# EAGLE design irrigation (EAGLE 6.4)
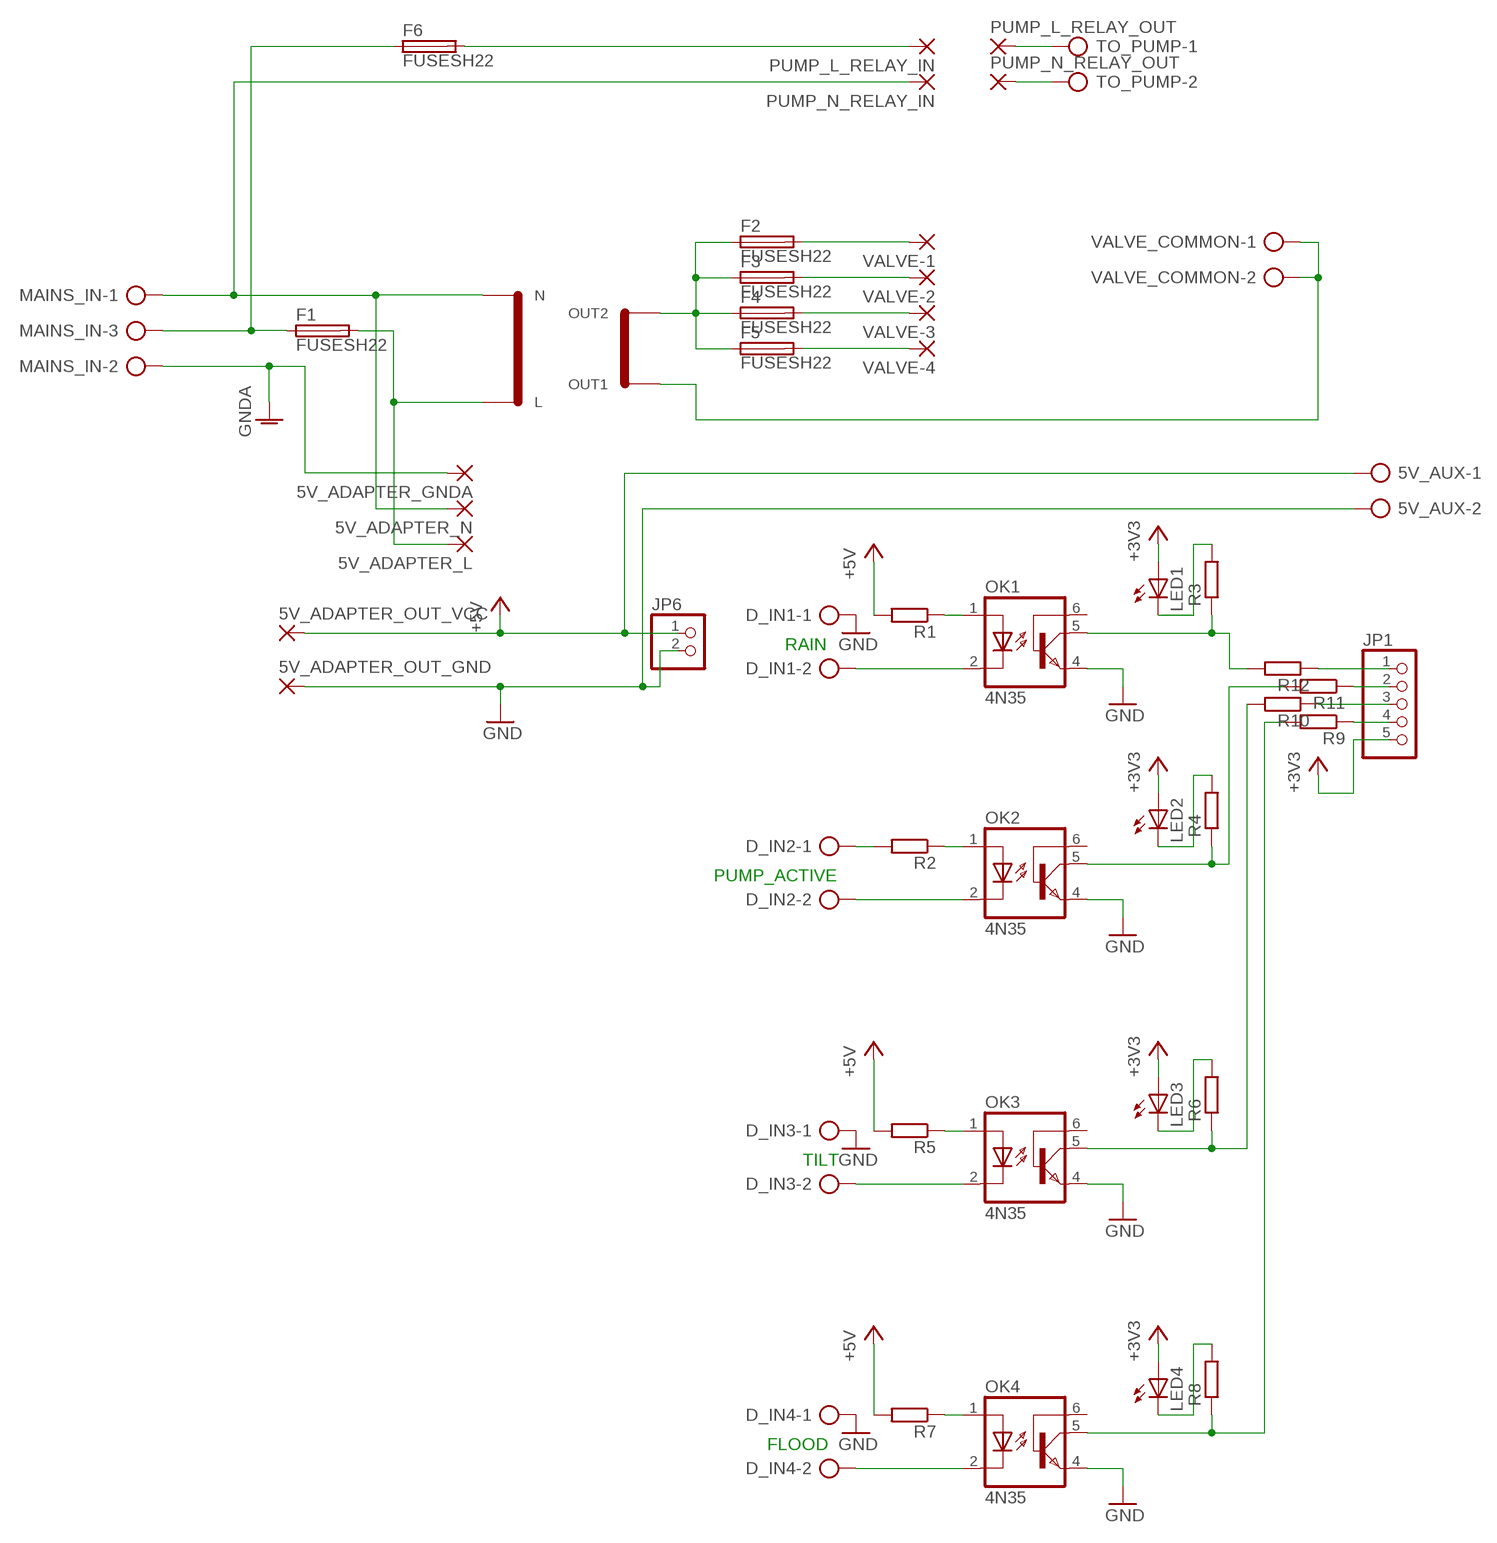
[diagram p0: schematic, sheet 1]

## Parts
5V_ADAPTER_GNDA  2,54/0,8  [2,54/0,8]
5V_ADAPTER_L  2,54/0,8  [2,54/0,8]
5V_ADAPTER_N  2,54/0,8  [2,54/0,8]
5V_ADAPTER_OUT_GND  2,54/0,8  [2,54/0,8]
5V_ADAPTER_OUT_VCC  2,54/0,8  [2,54/0,8]
5V_AUX  AK300/2  [AK300/2]
D_IN1  AK300/2  [AK300/2]
D_IN2  AK300/2  [AK300/2]
D_IN3  AK300/2  [AK300/2]
D_IN4  AK300/2  [AK300/2]
F1  FUSESH22  [SH22]
F2  FUSESH22  [SH22]
F3  FUSESH22  [SH22]
F4  FUSESH22  [SH22]
F5  FUSESH22  [SH22]
F6  FUSESH22  [SH22]
JP1  PINHD-1X5  [1X05]
JP6  PINHD-1X2  [1X02]
LED1  LED5MM  [LED5MM]
LED2  LED5MM  [LED5MM]
LED3  LED5MM  [LED5MM]
LED4  LED5MM  [LED5MM]
MAINS_IN  AK300/3  [AK300/3]
OK1  4N35  [DIL06]
OK2  4N35  [DIL06]
OK3  4N35  [DIL06]
OK4  4N35  [DIL06]
PUMP_L_RELAY_IN  2,54/0,8  [2,54/0,8]
PUMP_L_RELAY_OUT  2,54/0,8  [2,54/0,8]
PUMP_N_RELAY_IN  2,54/0,8  [2,54/0,8]
PUMP_N_RELAY_OUT  2,54/0,8  [2,54/0,8]
R1  R-EU_0207/10  [0207/10]
R2  R-EU_0207/10  [0207/10]
R3  R-EU_0207/10  [0207/10]
R4  R-EU_0207/10  [0207/10]
R5  R-EU_0207/10  [0207/10]
R6  R-EU_0207/10  [0207/10]
R7  R-EU_0207/10  [0207/10]
R8  R-EU_0207/10  [0207/10]
R9  R-EU_0207/10  [0207/10]
R10  R-EU_0207/10  [0207/10]
R11  R-EU_0207/10  [0207/10]
R12  R-EU_0207/10  [0207/10]
TO_PUMP  AK300/2  [AK300/2]
U$1  24V  [24V]
VALVE-1  2,54/0,8  [2,54/0,8]
VALVE-2  2,54/0,8  [2,54/0,8]
VALVE-3  2,54/0,8  [2,54/0,8]
VALVE-4  2,54/0,8  [2,54/0,8]
VALVE_COMMON  AK300/2  [AK300/2]

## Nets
+3V3: JP1.5 LED1.A LED2.A LED3.A LED4.A
+5V: 5V_ADAPTER_OUT_VCC.1(P) 5V_AUX.1 JP6.1 R1.2 R5.2 R7.2
GND: 5V_ADAPTER_OUT_GND.1(P) 5V_AUX.2 D_IN1.1 D_IN3.1 D_IN4.1 JP6.2 OK1.4(EMI) OK2.4(EMI) OK3.4(EMI) OK4.4(EMI)
MAINS_GNDA: 5V_ADAPTER_GNDA.1(P) MAINS_IN.2 ; supply symbol labelled GNDA
MAINS_L: F1.1 F6.1 MAINS_IN.3
MAINS_N: 5V_ADAPTER_N.1(P) MAINS_IN.1 PUMP_N_RELAY_IN.1(P) U$1.P$2(N)
N$1: F2.1 F3.1 F4.1 F5.1 U$1.P$4(OUT2)
N$2: JP1.1 R12.1
N$3: PUMP_N_RELAY_OUT.1(P) TO_PUMP.2
N$4: 5V_ADAPTER_L.1(P) F1.2 U$1.P$1(L)
N$5: LED2.K(C) R4.2
N$6: F2.2 VALVE-1.1(P)
N$7: F6.2 PUMP_L_RELAY_IN.1(P)
N$8: F3.2 VALVE-2.1(P)
N$9: PUMP_L_RELAY_OUT.1(P) TO_PUMP.1
N$10: F4.2 VALVE-3.1(P)
N$11: D_IN2.1 R2.2
N$12: F5.2 VALVE-4.1(P)
N$13: JP1.2 R11.1
N$14: JP1.3 R10.1
N$15: JP1.4 R9.1
N$17: LED1.K(C) R3.2
N$18: U$1.P$3(OUT1) VALVE_COMMON.1 VALVE_COMMON.2
N$19: OK2.5(COL) R4.1 R11.2
N$20: OK1.5(COL) R3.1 R12.2
N$21: OK1.1(A) R1.1
N$22: OK2.1(A) R2.1
N$23: D_IN1.2 OK1.2(C)
N$25: D_IN2.2 OK2.2(C)
N$28: LED3.K(C) R6.2
N$36: OK3.5(COL) R6.1 R10.2
N$41: OK3.1(A) R5.1
N$42: D_IN3.2 OK3.2(C)
N$44: LED4.K(C) R8.2
N$45: OK4.5(COL) R8.1 R9.2
N$46: OK4.1(A) R7.1
N$47: D_IN4.2 OK4.2(C)
Unconnected: OK1.6(BAS) OK2.6(BAS) OK3.6(BAS) OK4.6(BAS)

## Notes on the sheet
- RAIN
- PUMP_ACTIVE
- TILT
- FLOOD

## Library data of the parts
5V_ADAPTER_GNDA 5V_ADAPTER_L 5V_ADAPTER_N 5V_ADAPTER_OUT_GND 5V_ADAPTER_OUT_VCC PUMP_L_RELAY_IN PUMP_L_RELAY_OUT PUMP_N_RELAY_IN PUMP_N_RELAY_OUT VALVE-1-VALVE-4 = wirepad:2,54/0,8: THROUGH-HOLE PAD
5V_AUX D_IN1-D_IN4 TO_PUMP VALVE_COMMON = con-ptr500:AK300/2: CONNECTOR; OC_FARNELL: unknown; OC_NEWARK: unknown
F1-F6 = fuse:FUSE: Fuse; OC_FARNELL: unknown; OC_NEWARK: unknown
JP1 = pinhead:PINHD-1X5: PIN HEADER
JP6 = pinhead:PINHD-1X2: PIN HEADER
LED1-LED4 = led:LED: LED
MAINS_IN = con-ptr500:AK300/3: CONNECTOR; OC_FARNELL: unknown; OC_NEWARK: unknown
OK1-OK4 = optocoupler:4N35: MOTOROLA OPTO COUPLER; MF: FAIRCHILD SEMICONDUCTOR; MPN: 4N35; OC_FARNELL: 1328375; OC_NEWARK: 72K9946
R1-R12 = rcl:R-EU_: RESISTOR, European symbol
U$1 = jesiva_trafo:24V

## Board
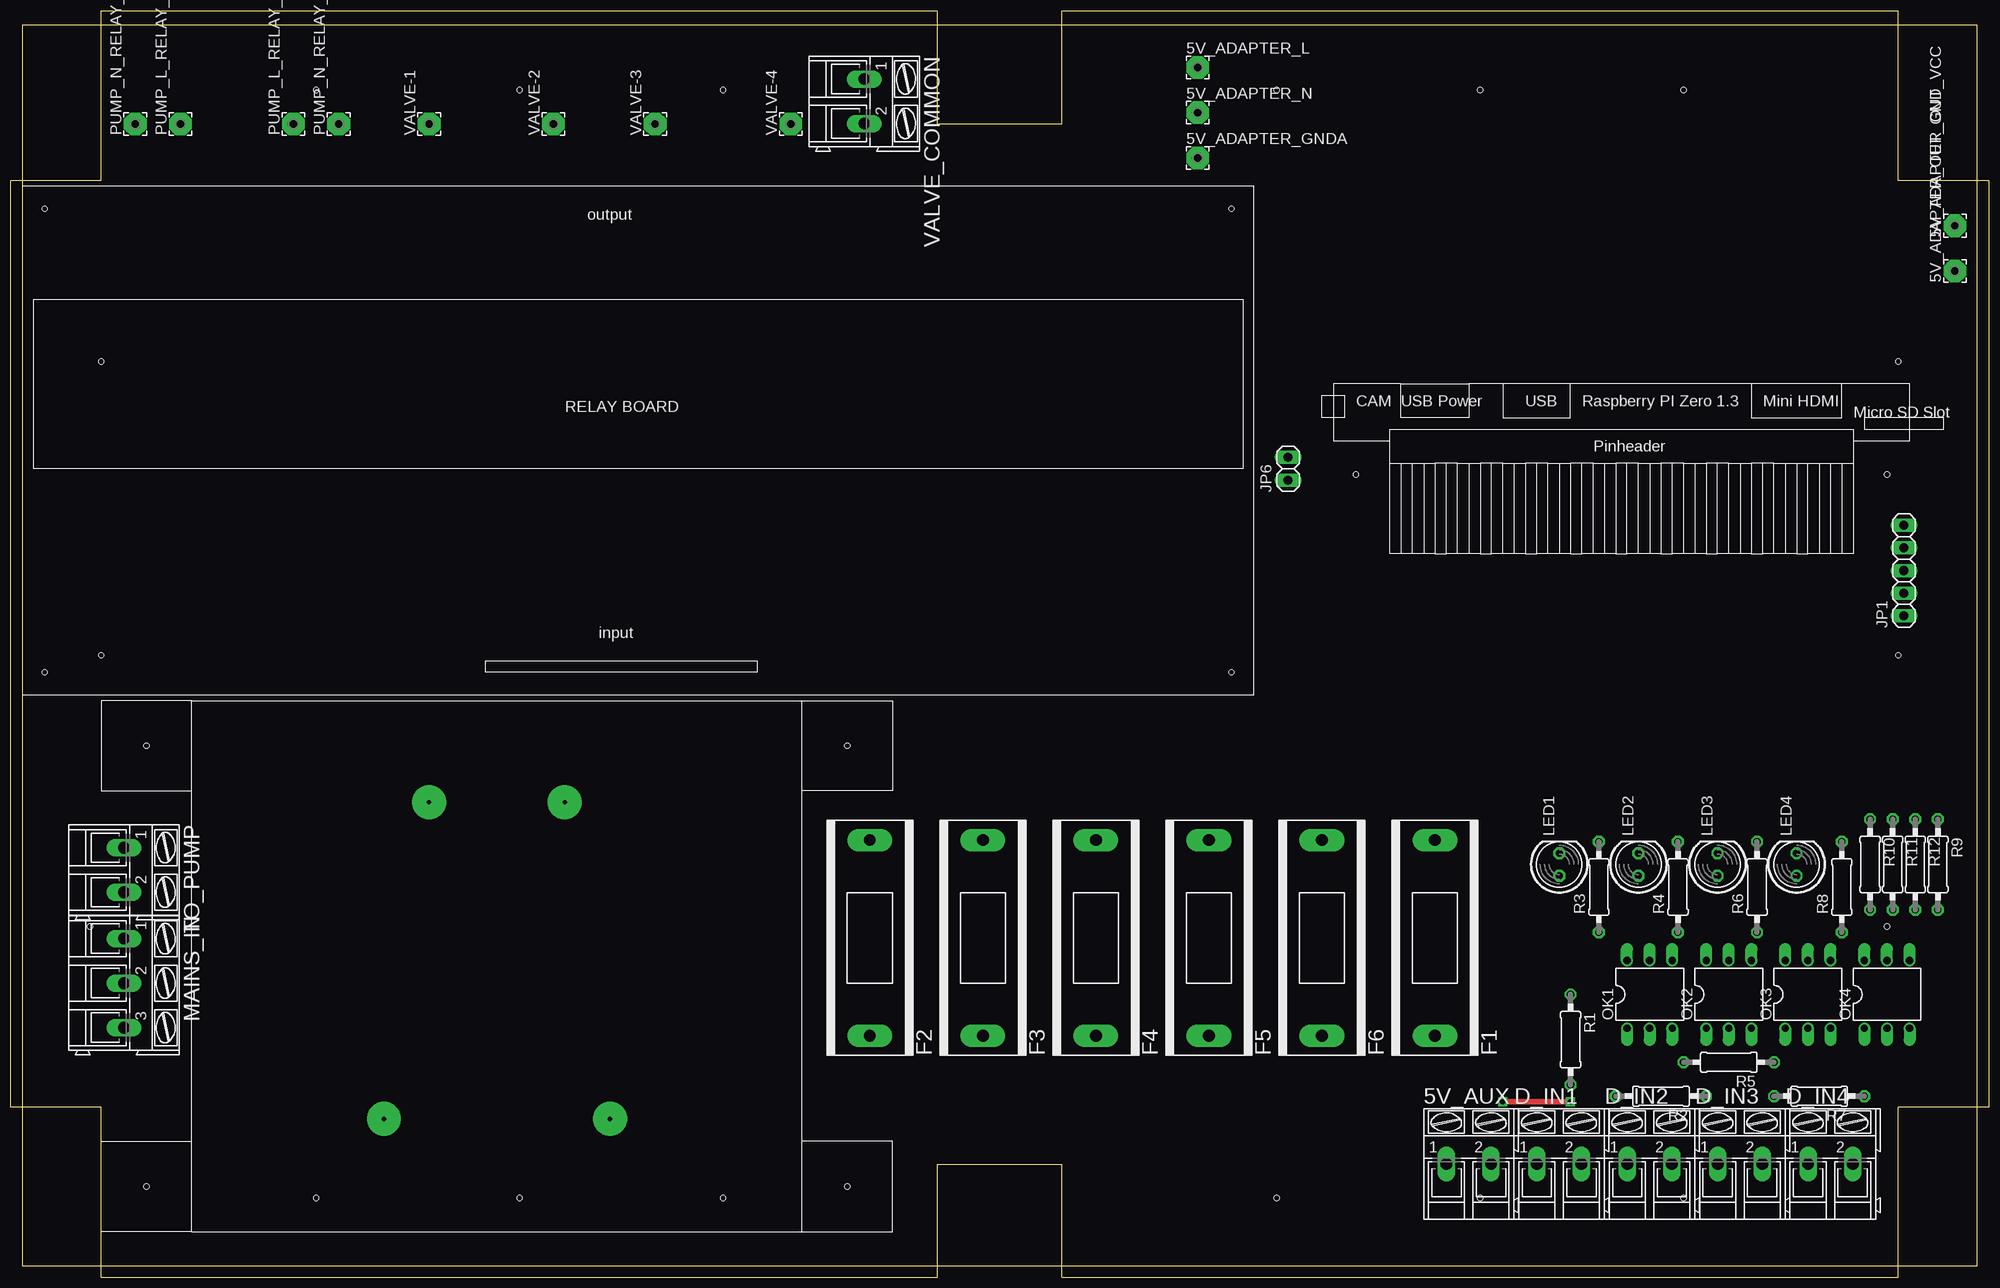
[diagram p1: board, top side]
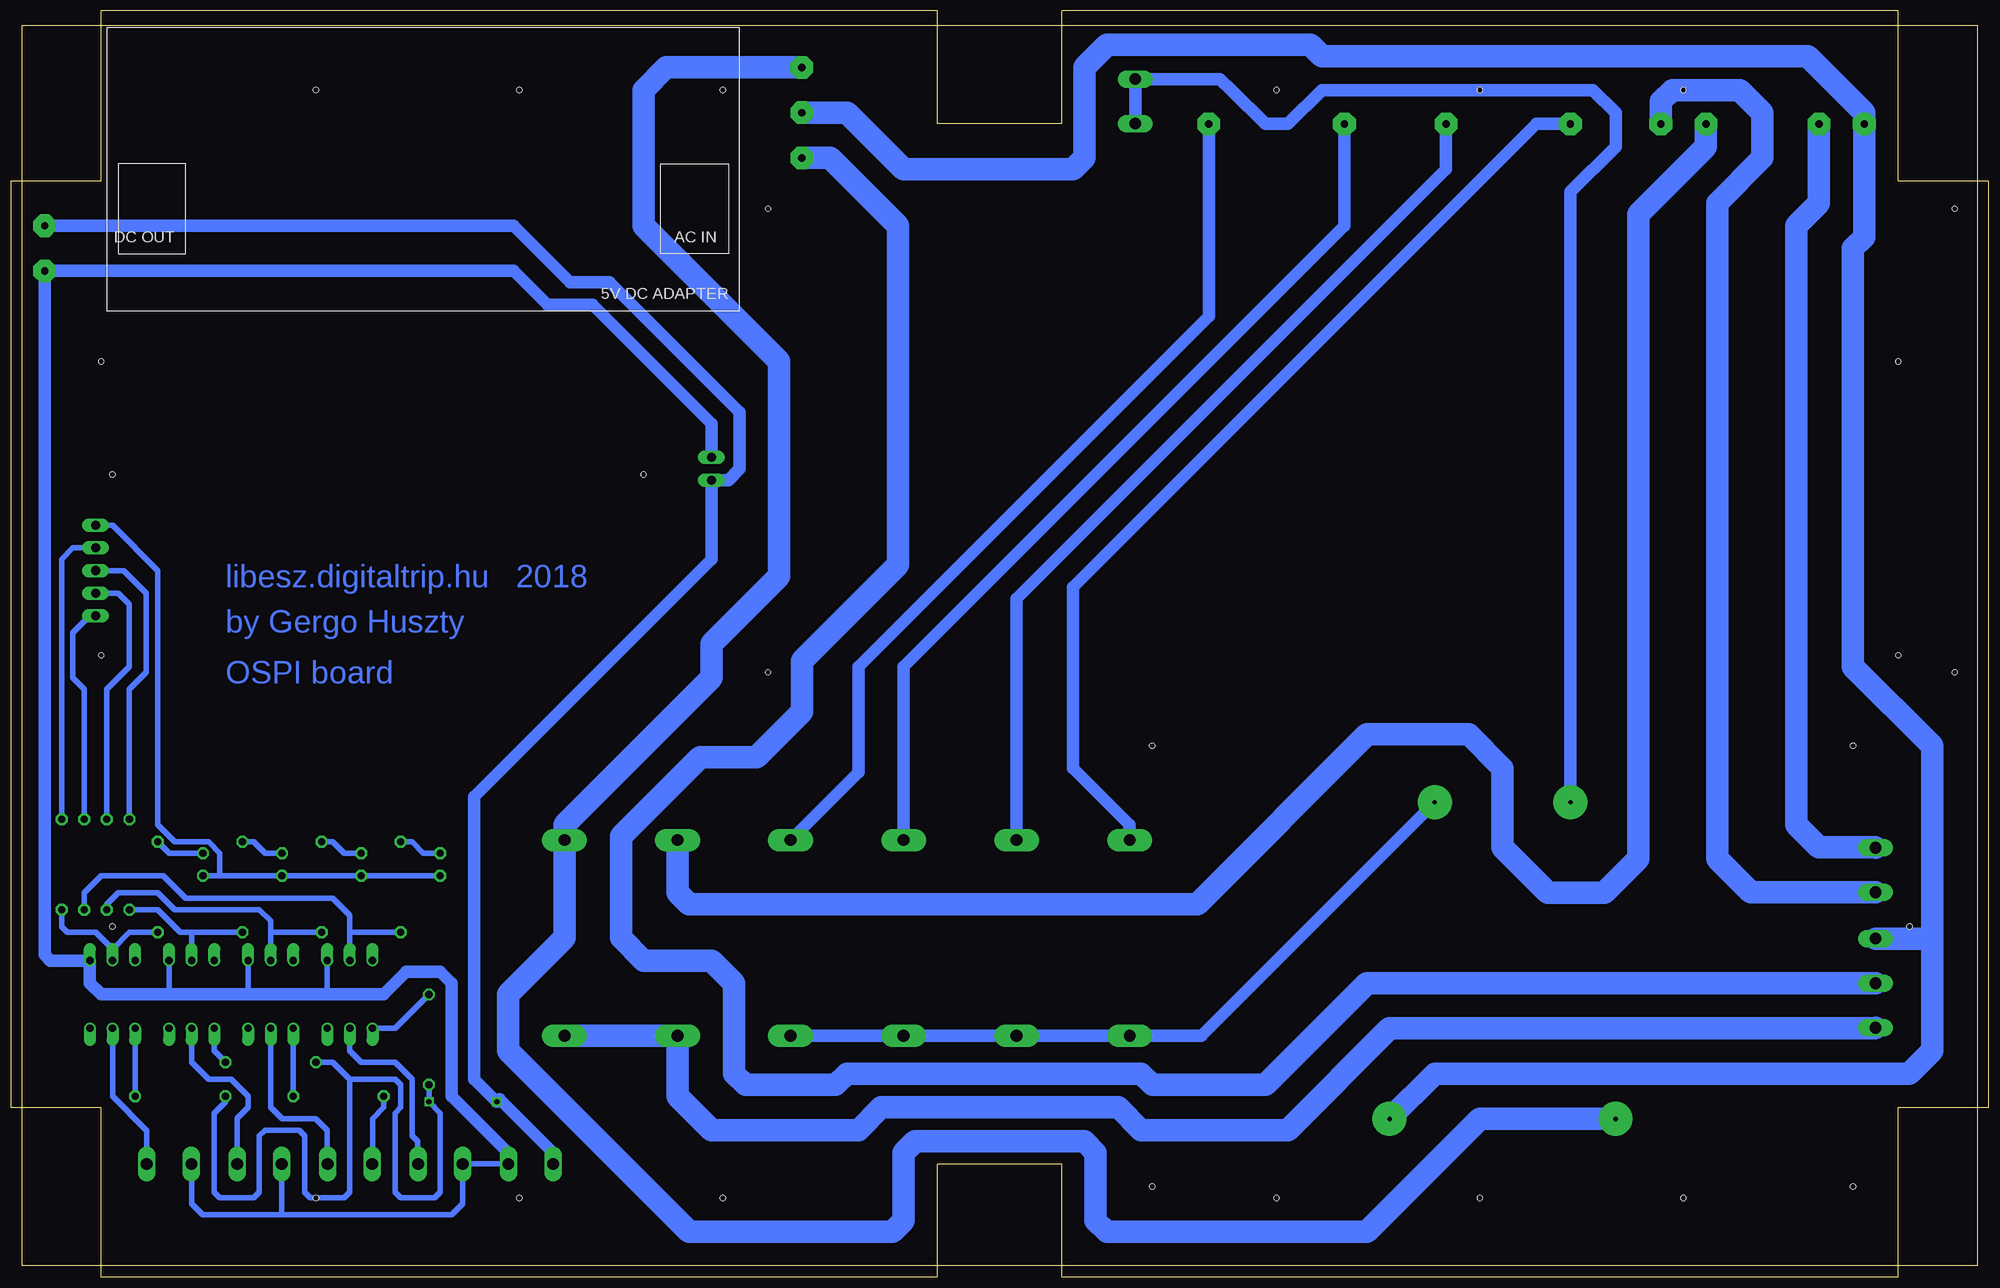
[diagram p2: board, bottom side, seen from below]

Size 219.69 x 139.37 mm. Coordinates in mm from the lower left corner, seen from the top.
Outline: 0,0 219.69,0 219.69,139.37 0,139.37 0,0
Copper layers (1*16): Top 0.035mm / dielectric 1.5mm / Bottom 0.035mm
Design rules "default": minimum track width 10mil, minimum drill 24mil, track to track 8mil, track to pad 8mil, pad to pad 8mil, via to via 8mil, smd to smd 8mil, copper to edge 40mil, drill to drill 8mil, minimum pad ring 10mil, minimum via ring 8mil, stop-mask expansion 4mil, vias tented up to drill 0mil, thermal gap 10mil

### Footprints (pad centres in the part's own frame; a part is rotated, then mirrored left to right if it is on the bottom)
2,54/0,8 = drill 0.813 pad 2.54 octagon: 1 0,0
AK300/2 = drill 1.321 long: 1 -2.515,0; 2 2.489,0
SH22 = drill 1.321 pad 2.54 long: 1 -10.998,0; 2 10.998,0
1X05 = drill 1.016 long: 1 -5.08,0; 2 -2.54,0; 3 0,0; 4 2.54,0; 5 5.08,0
1X02 = drill 1.016 long: 1 -1.27,0; 2 1.27,0
LED5MM = drill 0.813 octagon: A -1.27,0; K 1.27,0
AK300/3 = drill 1.321 long: 1 -5.004,0; 2 0,0; 3 5.004,0
DIL06 = drill 0.813 offset: 1 -2.54,-3.81; 2 0,-3.81; 3 2.54,-3.81; 4 2.54,3.81; 5 0,3.81; 6 -2.54,3.81
0207/10 = drill 0.813 octagon: 1 -5.08,0; 2 5.08,0
24V = drill 0.5 pad 3.81: P$1 0,25.4; P$2 0,0; P$3 35.56,20.32; P$4 35.56,5.08 | hole 0.6: -7.62,52.07; 41.91,52.07; 41.91,-26.67; -7.62,-26.67
RASPBERRY_PI_ZERO_ON_EDGE = hole 0.6: 2.54,-10.16; 62.23,-10.16
PROJECT_BOX = hole 0.6: 191.77,137.16; 168.91,137.16; 146.05,137.16; 83.82,137.16; 60.96,137.16; 38.1,137.16; 83.82,12.7; 60.96,12.7; 38.1,12.7; 191.77,12.7; 168.91,12.7; 146.05,12.7; 215.9,106.68; 215.9,73.66; 214.63,43.18; 13.97,106.68; 13.97,73.66; 12.7,43.18
RELAY_BOARD_8 = hole 0.6: 2.54,2.54; 2.54,54.61; 135.89,54.61; 135.89,2.54

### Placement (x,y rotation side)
5V_ADAPTER_GNDA  132.08,124.46 0 top
5V_ADAPTER_L  132.08,134.62 0 top
5V_ADAPTER_N  132.08,129.54 0 top
5V_ADAPTER_OUT_GND  217.17,111.76 90 top
5V_ADAPTER_OUT_VCC  217.17,116.84 90 top
5V_AUX  162.56,11.43 0 top
D_IN1  172.72,11.43 0 top
D_IN2  182.88,11.43 0 top
D_IN3  193.04,11.43 0 top
D_IN4  203.2,11.43 0 top
F1  158.75,36.83 90 top
F2  95.25,36.83 90 top
F3  107.95,36.83 90 top
F4  120.65,36.83 90 top
F5  133.35,36.83 90 top
F6  146.05,36.83 90 top
JP1  211.46,78.11 90 top
JP6  142.24,89.53 90 top
LED1  172.72,45.09 90 top
LED2  181.61,45.09 90 top
LED3  190.5,45.09 90 top
LED4  199.39,45.09 90 top
MAINS_IN  11.43,31.75 270 top
OK1  182.88,30.48 0 top
OK2  191.77,30.48 0 top
OK3  200.66,30.48 0 top
OK4  209.55,30.48 0 top
PUMP_L_RELAY_IN  30.48,128.27 90 top
PUMP_L_RELAY_OUT  17.78,128.27 90 top
PUMP_N_RELAY_IN  12.7,128.27 90 top
PUMP_N_RELAY_OUT  35.56,128.27 90 top
R1  173.99,25.4 270 top
R2  184.15,19.05 180 top
R3  177.17,42.55 90 top
R4  186.06,42.55 90 top
R5  191.77,22.86 180 top
R6  194.95,42.55 90 top
R7  201.93,19.05 180 top
R8  204.47,42.55 90 top
R9  215.27,45.09 270 top
R10  207.65,45.09 270 top
R11  210.19,45.09 270 top
R12  212.73,45.09 270 top
TO_PUMP  11.43,44.45 270 top
U$1  66.04,16.51 90 top
U$2  [RASPBERRY_PI_ZERO_ON_EDGE]  147.32,99.06 0 top
U$3  [PROJECT_BOX]  -5.08,-5.08 0 top
U$4  [RELAY_BOARD_8]  0,64.14 0 top
U$5  [5V_ADAPTER_ON_EDGE]  139.06,139.06 180 bottom
VALVE-1  45.72,128.27 90 top
VALVE-2  59.69,128.27 90 top
VALVE-3  71.12,128.27 90 top
VALVE-4  86.36,128.27 90 top
VALVE_COMMON  94.61,130.81 270 top

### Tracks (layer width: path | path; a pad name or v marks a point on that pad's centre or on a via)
+3V3
  Bottom 0.61: LED1.A LED2.A LED3.A 197.49,43.81 | 197.49,43.81 LED4.A | 197.49,43.81 197.49,46.35 198.76,47.62 202.56,47.62 204.47,49.53 204.47,78.11 209.55,83.19 JP1.5
+5V  (via drill 0.6)
  Top 0.61: v173.99,18.41 v166.37,18.41
  Bottom 0.61: 160.02,11.4 5V_AUX.1 | R7.2 196.85,18.41 198.12,17.14 198.12,8.26 197.49,7.62 193.68,7.62 193.04,8.26 193.04,14.61 192.41,15.24 188.59,15.24 187.96,14.61 187.96,8.26 187.33,7.62 183.52,7.62 182.88,8.26 182.88,20.95 | v166.37,18.41 166.05,18.73 | R1.2 v173.99,18.41 172.72,17.14 172.72,8.26 173.36,7.62 177.17,7.62 177.8,8.26 177.8,17.14 177.17,17.78 177.17,20.32 177.8,20.95 182.88,20.95 | 182.88,20.95 184.78,22.86 R5.2
  Bottom 1.27: 160.02,11.46 5V_AUX.1
  Bottom 1.422: 160.02,11.46 160.02,12.7 166.05,18.73 | 5V_ADAPTER_OUT_VCC.1 164.47,116.84 158.12,110.49 153.67,110.49 139.06,95.89 139.06,89.53 140.34,88.27 JP6.1 142.24,79.38 168.91,52.7 168.91,20.95 v166.37,18.41
GND
  Bottom 0.61: 194.31,30.48 OK2.4 | OK1.4 185.42,30.48 | OK3.4 203.2,30.48 | 165.1,11.48 170.16,11.48 D_IN1.1 170.21,6.96 171.45,5.71 180.34,5.71 | 180.34,5.71 190.5,5.71 | 190.5,5.71 199.39,5.71 200.66,6.99 200.66,11.4 D_IN4.1 | D_IN3.1 190.53,5.74 190.5,5.71 | 180.37,5.74 180.34,5.71
  Bottom 1.422: 5V_AUX.2 165.1,11.48 165.1,12.7 171.45,19.05 171.45,31.75 172.72,33.02 176.53,33.02 179.07,30.48 185.42,30.48 194.31,30.48 203.2,30.48 210.82,30.48 212.09,31.75 OK4.4 216.53,34.29 217.17,34.92 5V_ADAPTER_OUT_GND.1 164.47,111.76 160.66,107.95 155.58,107.95 142.24,94.61 JP6.2
MAINS_GNDA
  Bottom 2.54: 5V_ADAPTER_GNDA.1 128.91,124.46 121.28,116.84 121.28,78.74 132.08,67.94 132.08,62.23 137.16,57.15 143.51,57.15 152.4,48.26 152.4,36.83 149.86,34.29 142.24,34.29 139.7,31.75 139.7,21.59 138.43,20.32 128.27,20.32 127,21.59 93.98,21.59 92.71,20.32 80.01,20.32 68.58,31.75 MAINS_IN.2
MAINS_L
  Bottom 2.54: F1.1 F6.1 146.05,19.05 142.24,15.24 125.73,15.24 123.19,17.78 96.52,17.78 93.98,15.24 77.47,15.24 66.04,26.67 11.51,26.67 MAINS_IN.3
MAINS_N
  Bottom 2.54: U$1.P$2 60.96,21.59 7.62,21.59 5.08,24.13 5.08,36.83 | 5.08,36.83 5.08,58.42 13.97,67.31 13.97,114.3 12.7,115.57 PUMP_N_RELAY_IN.1 12.7,129.54 19.05,135.89 73.66,135.89 74.93,137.16 97.79,137.16 100.33,134.62 100.33,124.46 101.6,123.19 120.65,123.19 127,129.54 5V_ADAPTER_N.1 | MAINS_IN.1 5.16,36.75 5.08,36.83
N$1
  Bottom 1.422: F5.1 121.08,25.83 120.65,25.4 F4.1 F3.1 F2.1 87.2,25.83 U$1.P$4
N$2
  Bottom 0.61: R12.1 212.73,64.77 214,66.04 214,71.12 212.09,73.03 JP1.1
N$3
  Bottom 2.54: PUMP_N_RELAY_OUT.1 35.56,130.81 34.29,132.08 26.67,132.08 24.13,129.54 24.13,124.46 29.21,119.38 29.21,45.72 25.45,41.96 TO_PUMP.2
N$4
  Bottom 2.54: U$1.P$1 55.88,16.51 68.58,3.81 97.79,3.81 99.06,5.08 99.06,12.7 100.33,13.97 119.38,13.97 120.65,12.7 120.65,5.08 121.92,3.81 144.78,3.81 165.1,24.13 165.1,30.48 158.75,36.83 F1.2 158.75,49.53 142.24,66.04 142.24,69.85 134.62,77.47 134.62,101.6 149.86,116.84 149.86,132.08 147.32,134.62 5V_ADAPTER_L.1
N$5
  Bottom 0.61: LED2.K 183.52,46.35 184.78,47.62 R4.2
N$6
  Bottom 1.422: F2.2 95.25,49.53 101.6,55.88 101.6,76.2 49.53,128.27 VALVE-1.1
N$7
  Bottom 2.54: F6.2 146.05,41.91 144.78,40.64 87.63,40.64 68.58,59.69 57.15,59.69 53.34,55.88 53.34,46.99 48.26,41.91 41.91,41.91 38.1,45.72 38.1,118.11 30.48,125.73 PUMP_L_RELAY_IN.1
N$8
  Bottom 1.422: F3.2 107.95,74.93 59.69,123.19 VALVE-2.1
N$9
  Bottom 2.54: PUMP_L_RELAY_OUT.1 17.78,119.38 20.32,116.84 20.32,49.53 17.78,46.99 11.46,46.99 TO_PUMP.1
N$10
  Bottom 1.422: F4.2 120.65,67.31 71.12,116.84 VALVE-3.1
N$11
  Bottom 0.406: 180.34,11.46 D_IN2.1
  Bottom 0.61: R2.2 179.07,17.78 180.34,16.51 180.34,11.46
N$12
  Bottom 1.422: VALVE-4.1 86.36,106.68 125.73,67.31 125.73,55.45 F5.2
N$13
  Bottom 0.61: R11.1 210.19,64.77 207.65,67.31 207.65,74.3 208.92,75.56 JP1.2
N$14
  Bottom 0.61: R10.1 207.65,64.77 205.74,66.67 205.74,75.56 208.28,78.11 JP1.3
N$15
  Bottom 0.61: R9.1 215.27,79.38 214,80.64 JP1.4
N$17
  Bottom 0.61: LED1.K 174.62,46.35 175.9,47.62 R3.2
N$18
  Bottom 1.422: VALVE_COMMON.2 VALVE_COMMON.1 85.11,133.32 83.82,132.08 80.01,128.27 77.47,128.27 73.66,132.08 43.18,132.08 40.64,129.54 40.64,125.73 45.72,120.65 U$1.P$3
N$19
  Bottom 0.61: 191.77,37.47 191.77,38.73 193.04,40.01 202.56,40.01 204.47,41.91 208.92,41.91 210.19,40.64 R11.2 | 191.77,37.47 OK2.5 | R4.1 191.77,37.47
N$20
  Bottom 0.61: OK1.5 182.88,37.47 | 182.88,37.47 182.88,39.37 184.78,41.27 201.3,41.27 203.84,43.81 210.82,43.81 212.73,41.91 R12.2 | R3.1 182.88,37.47
N$21
  Bottom 0.61: OK1.1 177.8,26.67 R1.1
N$22
  Bottom 0.61: OK2.1 R2.1
N$23
  Bottom 0.61: OK1.2 182.88,24.13 181.61,22.86 177.8,22.86 175.9,20.95 175.9,14.61 175.26,13.97 175.26,11.48 D_IN1.2
N$25
  Bottom 0.61: OK2.2 191.77,17.78 190.5,16.51 186.69,16.51 185.42,15.24 185.42,11.48 D_IN2.2
N$28
  Bottom 0.61: LED3.K 192.41,46.35 193.68,47.62 R6.2
N$36
  Bottom 0.61: 200.66,37.47 OK3.5 | R6.1 200.66,37.47 | 200.66,37.47 201.93,37.47 204.47,40.01 R10.2
N$41
  Bottom 0.61: OK3.1 198.12,24.13 R5.1
N$42
  Bottom 0.61: 200.61,26.62 OK3.2 200.66,22.86 198.76,20.95 196.22,20.95 194.31,19.05 194.31,17.78 195.53,16.56 D_IN3.2
N$44
  Bottom 0.61: LED4.K 203.2,46.35 R8.2
N$45
  Bottom 0.61: 209.55,35.56 OK4.5 | R8.1 207.65,37.47 209.55,35.56 | R9.2 215.27,38.1 214.63,37.47 211.46,37.47 209.55,35.56
N$46
  Bottom 0.61: OK4.1 R7.1
N$47
  Bottom 0.61: D_IN4.2 205.69,15.19 209.55,19.05 OK4.2

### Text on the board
Bottom: libesz.digitaltrip.hu 2018 | by Gergo Huszty | OSPI board
Document: OSPi - Modified by Gergo Huszty - 2017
